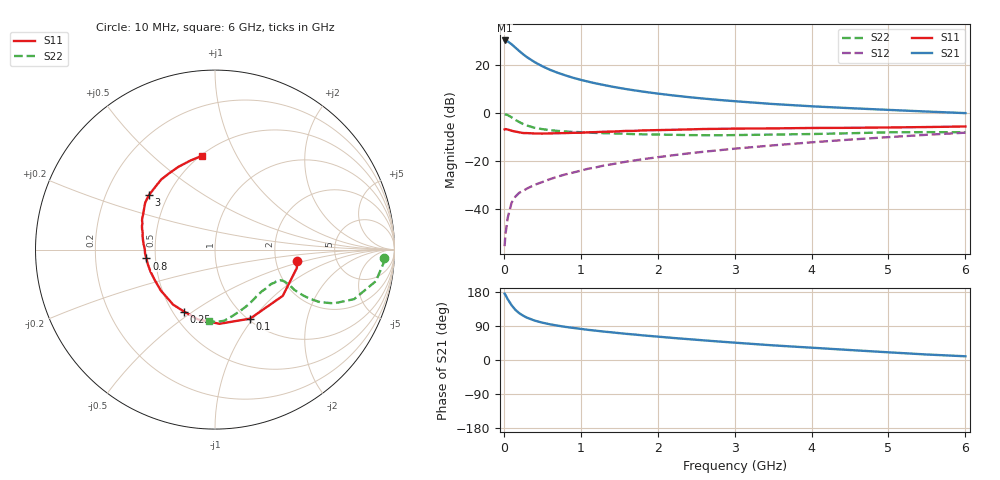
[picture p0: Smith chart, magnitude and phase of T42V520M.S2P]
! Infineon Technologies  Discrete & RF Semiconductors
! BFR182T
! Si NPN RF Bipolar Junction Transistor in SC75
! VCE = 2.5 V  IC = 20 mA
! Common Emitter S-Parameters:  October  1999
# GHz  S  MA  R  50
!  f  S11  S21  S12  S22
! GHz  MAG  ANG  MAG  ANG  MAG  ANG  MAG  ANG
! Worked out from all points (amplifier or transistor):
!   36 points, 10 MHz to 6 GHz, reference 50 ohm
!   highest |S21| = 30.3 dB at 10 MHz (marker M1)
!   |S21| within 3 dB of that: start of sweep to 150.7 MHz
!   unconditionally stable (mu >= 1): 561.5 MHz to 3.737 GHz
!   at 250 MHz: K = 0.69, MSG = 28.5 dB, |S12| = -32.4 dB
!   at 1.4 GHz: K = 1.14, MAG = 13.9 dB, |S12| = -21.3 dB
!   at 6 GHz: K = 0.85, MSG = 4.1 dB, |S12| = -8.1 dB
!   S11 on the Smith chart (normalised r, x): 10 MHz: 2.62, -0.43; 100 MHz: 1.02, -0.97; 250 MHz: 0.57, -0.46; 800 MHz: 0.44, -0.05; 3 GHz: 0.39, +0.31; 6 GHz: 0.51, +0.74
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0.01  0.4592 -8.1  32.74 175.0  0.0017 80.2  0.9437 -2.9
0.02  0.4675 -12.6  32.54 172.2  0.0029 83.3  0.9424 -4.5
0.05  0.4572 -34.3  31.31 160.6  0.0066 84.5  0.9134 -11.1
0.1  0.4315 -63.1  27.38 144.7  0.0136 71.0  0.8227 -19.6
0.15  0.414 -86.5  23.23 132.4  0.0183 66.0  0.7278 -24.3
0.2  0.4005 -103.5  19.75 123.6  0.022 63.7  0.6548 -26.6
0.25  0.3862 -116.5  16.93 117.0  0.0241 62.3  0.5951 -27.4
0.3  0.385 -127.3  14.71 111.8  0.0269 63.4  0.5543 -27.5
0.4  0.3784 -142.8  11.6 104.0  0.0322 63.7  0.4963 -26.9
0.5  0.3762 -153.1  9.506 98.6  0.0368 65.0  0.4658 -25.7
0.6  0.3796 -161.0  8.014 94.2  0.0423 67.1  0.4435 -25.1
0.8  0.3857 -172.7  6.134 87.4  0.0531 68.9  0.4159 -24.7
0.9  0.3904 -177.2  5.471 84.7  0.058 70.3  0.4065 -24.9
1.1  0.3997 175.3  4.524 79.5  0.0699 70.9  0.395 -25.9
1.3  0.411 169.2  3.862 75.0  0.0813 71.6  0.3834 -27.5
1.6  0.4283 161.9  3.16 68.9  0.0983 71.4  0.3713 -30.4
2.2  0.4512 151.7  2.345 58.2  0.133 70.9  0.3549 -38.5
3  0.477 140.5  1.778 45.8  0.1825 68.3  0.35 -50.2
3.5  0.4825 133.6  1.553 38.6  0.2138 66.2  0.3587 -58.6
4.5  0.4959 121.2  1.273 26.3  0.2818 60.8  0.3822 -75.0
5.5  0.5149 105.3  1.082 14.5  0.3552 54.3  0.4031 -89.0
6  0.5286 97.6  1.004 9.8  0.3931 50.3  0.4008 -94.9
